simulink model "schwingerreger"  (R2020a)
settings: Solver=ode45  StartTime=0.0  StopTime=10  RelTol=1e-3  EnableMultiTasking=on

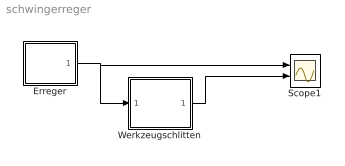
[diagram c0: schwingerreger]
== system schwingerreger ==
  Erreger : Subsystem
  Scope1 : Scope  NumInputPorts=2
  Werkzeugschlitten : Subsystem  mask(Schwingkreis){D=0.001, om0=50, b0=40}
      mask prompts: D "Daempfungsgrad"; om0 "Eigenfrequenz"; b0 "Staerke"
      mask help: Harmonischer Schwinger mit Eigenfrequenz omega0 und Daempfungsgrad D. Die Erregerfunktion werde mit einer Verstaerkung eingekoppelt.
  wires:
  Erreger/1(Out) -> Werkzeugschlitten/1(u), Scope1/1
  Werkzeugschlitten/1(x) -> Scope1/2

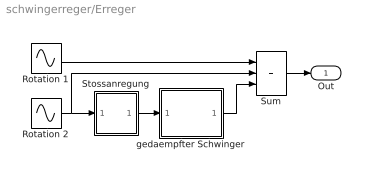
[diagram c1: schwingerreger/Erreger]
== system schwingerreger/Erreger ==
  Rotation 1 : Sin  Amplitude=2  Frequency=8  SampleTime=0
  Rotation 2 : Sin  Amplitude=4  Frequency=2  SampleTime=0
  Stossanregung : Subsystem  mask(Stossanregung){startlevel=2, stoplevel=2.1, amplitude=2}
      mask help: erzeugt aus Sinus periodischen Rechteckimpuls
  Sum : Sum  Inputs=+++  SaturateOnIntegerOverflow=on
  gedaempfter Schwinger : Subsystem  mask(Schwingkreis){D=0.025, om0=50, b0=400}
      mask prompts: D "Daempfungsgrad"; om0 "Eigenfrequenz"; b0 "Staerke"
      mask help: Harmonischer Schwinger mit Eigenfrequenz omega0 und Daempfungsgrad D. Die Erregerfunktion werde mit einer Verstaerkung eingekoppelt.
  Out : Outport
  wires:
  Rotation 2/1 -> Stossanregung/1(In1), Sum/2
  Sum/1 -> Out/1
  Stossanregung/1(Out1) -> gedaempfter Schwinger/1(u)
  Rotation 1/1 -> Sum/1
  gedaempfter Schwinger/1(x) -> Sum/3

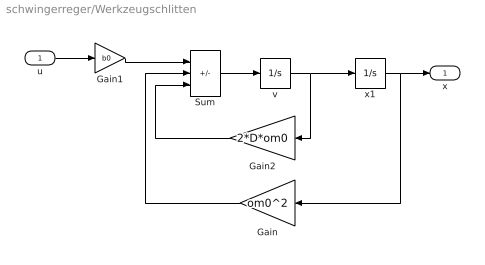
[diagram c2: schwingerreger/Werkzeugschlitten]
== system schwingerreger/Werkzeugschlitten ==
  u : Inport
  Gain : Gain  Gain=om0^2  SaturateOnIntegerOverflow=on
  Gain1 : Gain  Gain=b0  SaturateOnIntegerOverflow=on
  Gain2 : Gain  Gain=2*D*om0  SaturateOnIntegerOverflow=on
  Sum : Sum  Inputs=+--  SaturateOnIntegerOverflow=on
  v : Integrator
  x1 : Integrator
  x : Outport
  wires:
  Sum/1 -> v/1
  v/1 -> x1/1, Gain2/1
  Gain1/1 -> Sum/1
  x1/1 -> x/1, Gain/1
  u/1 -> Gain1/1
  Gain2/1 -> Sum/3
  Gain/1 -> Sum/2

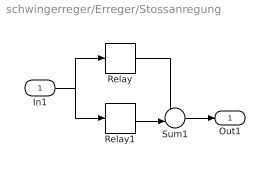
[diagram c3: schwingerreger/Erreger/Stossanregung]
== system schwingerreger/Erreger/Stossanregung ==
  In1 : Inport
  Relay : Relay  OnSwitchValue=startlevel  OffSwitchValue=0  OnOutputValue=amplitude
  Relay1 : Relay  OnSwitchValue=stoplevel  OffSwitchValue=0  OnOutputValue=amplitude
  Sum1 : Sum  Inputs=+-|  SaturateOnIntegerOverflow=on
  Out1 : Outport
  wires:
  Relay/1 -> Sum1/1
  Relay1/1 -> Sum1/2
  In1/1 -> Relay/1, Relay1/1
  Sum1/1 -> Out1/1

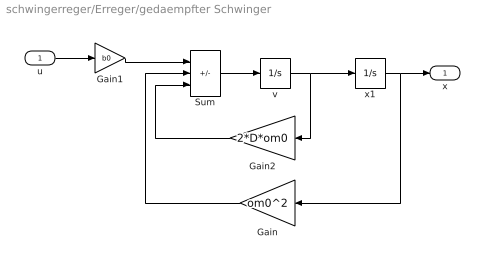
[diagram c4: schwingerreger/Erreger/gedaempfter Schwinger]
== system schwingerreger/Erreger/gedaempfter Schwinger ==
  u : Inport
  Gain : Gain  Gain=om0^2  SaturateOnIntegerOverflow=on
  Gain1 : Gain  Gain=b0  SaturateOnIntegerOverflow=on
  Gain2 : Gain  Gain=2*D*om0  SaturateOnIntegerOverflow=on
  Sum : Sum  Inputs=+--  SaturateOnIntegerOverflow=on
  v : Integrator
  x1 : Integrator
  x : Outport
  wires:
  Gain/1 -> Sum/2
  Gain2/1 -> Sum/3
  u/1 -> Gain1/1
  x1/1 -> Gain/1, x/1
  Gain1/1 -> Sum/1
  v/1 -> Gain2/1, x1/1
  Sum/1 -> v/1
